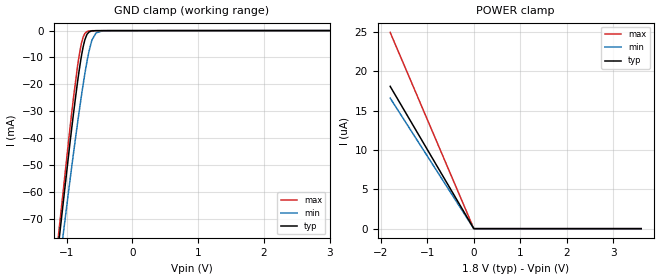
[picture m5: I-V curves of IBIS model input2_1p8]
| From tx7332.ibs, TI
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|   input2_1p8 Model
[Model]   input2_1p8
Model_type   Input
Vinl = 0.45
Vinh = 1.35
|   typ   min   max
C_comp   3.174pF   3.174pF   3.204pF
[Model spec]
|subparameter
Vinl   0.45   0.425   0.475
Vinh   1.35   1.275   1.425
| Where Nom  PVT is Nominal Process, 1.8V, 27C
|   Fast PVT is Strong Process,  1.9V, 0C
|   Slow PVT is Weak Process,   1.7V, 100C
[Voltage Range]   1.8   1.7   1.9
|Junction Temperature
[Temperature Range]   27   100   0
[Power Clamp Reference]   1.8   1.7   1.9
[GND Clamp Reference]   0   0   0
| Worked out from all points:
|   GND clamp passes 1 mA (typ) near -0.68 V on its own axis
[GND Clamp]
|   Voltage   I(typ)   I(min)   I(max)
-1.8V     -235.4mA   -228.3mA   -240.4mA
-1.136V   -82.24mA   -92.1mA    -78.7mA
-957.6mV  -43.46mA   -57.23mA   -37.99mA
-892.8mV  -30.21mA   -45.03mA   -24.32mA
-828mV    -17.96mA   -33.27mA   -12.19mA
-784.8mV  -10.84mA   -25.82mA   -5.841mA
-752.4mV  -6.425mA   -20.51mA   -2.645mA
-693mV    -1.523mA   -11.75mA   -388.8uA
-612mV    -116.2uA   -3.371mA   -54.47uA
-552.6mV  -33.93uA   -832.4uA   -36.76uA
-444.6mV  -22.7uA    -55.7uA    -32.51uA
3.6V      0A         0A         0A
[POWER Clamp]
|   Voltage   I(typ)   I(min)   I(max)
-1.8V     18.07uA    16.58uA    24.92uA
-7.2mV    54.44nA    48.69nA    81.99nA
-1.8mV    305.4pA    24.34nA    7.212nA
3.6V      0A         0A         0A
